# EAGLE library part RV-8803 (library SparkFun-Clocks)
Micro Crystal RV-8803 - Temperature compensated RTC Ultra accurate plus/minus 3PPM I2C RTC. Temperature compensated crystal for low drift
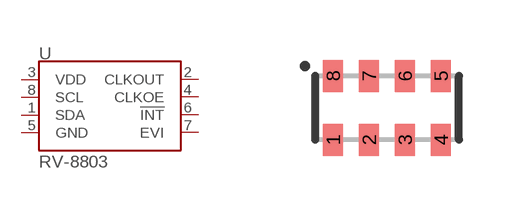
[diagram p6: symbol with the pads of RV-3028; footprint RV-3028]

Designator prefix U

## RV-8803 (PROD_ID: IC-14828; VALUE: RV-8803)  [RV-3028]
1  SDA
2  CLKOUT
3  VDD
4  CLKOE
5  GND
6  !INT
7  EVI
8  SCL

## Footprint RV-3028 (pad centres in mm)
Footprint for the RV-3028 I2C RTC
smd 0.5 x 0.8: 1 -1.35,-0.8; 2 -0.45,-0.8; 3 0.45,-0.8; 4 1.35,-0.8; 5 1.35,0.8; 6 0.45,0.8; 7 -0.45,0.8; 8 -1.35,0.8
